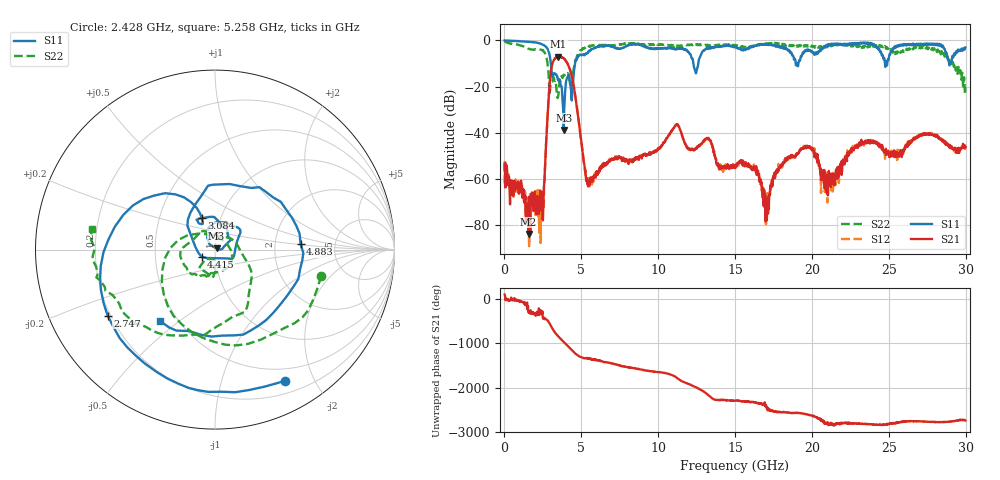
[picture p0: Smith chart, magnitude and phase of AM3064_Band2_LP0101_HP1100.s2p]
# Hz S DB R 50.0
!freq dBS11 angS11 dBS21 angS21 dBS12 angS12 dBS22 angS22
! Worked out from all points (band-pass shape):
!   1600 points, 10 MHz to 29.98 GHz, reference 50 ohm
!   highest |S21| = -7.01 dB at 3.515 GHz (marker M1); lowest = -83.8 dB at 1.566 GHz (marker M2)
!   |S21| within 3 dB of the highest: 3.122 GHz to 4.094 GHz (972 MHz wide, 26.9 % of centre)
!   lowest |S11| = -38.7 dB at 3.852 GHz (marker M3), VSWR 1.02, Z = 50.9 + j0.73 ohm
!   |S11| at or under -10 dB: 3.019 GHz to 4.593 GHz (1.574 GHz wide, 41.4 % of centre); 12.29 GHz to 12.61 GHz (322.1 MHz wide, 2.59 % of centre); 18.95 GHz to 19.12 GHz (176.6 MHz wide, 0.928 % of centre)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
!   |S22| runs from -25.0 to -0.3 dB; largest |S21 - S12| = 0.011
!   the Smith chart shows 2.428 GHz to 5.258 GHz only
!   S11 on the Smith chart (normalised r, x): 2.428 GHz: 0.35, -1.62; 2.747 GHz: 0.19, -0.27; 3.084 GHz: 0.82, +0.30; 4.415 GHz: 0.86, -0.07; 4.883 GHz: 2.81, +0.23; 5.258 GHz: 0.40, -0.43
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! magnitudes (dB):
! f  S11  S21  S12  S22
! 10 MHz  0.0  -53.7  -52.4  -0.3
! 1.566 GHz  -0.6  -83.8  -77.2  -3.6
! 2.428 GHz  -1.6  -65.5  -71.9  -4.3
! 2.747 GHz  -3.1  -40.0  -39.9  -7.7
! 3.084 GHz  -14.5  -10.8  -10.8  -18.0
! 3.515 GHz  -17.3  -7.0  -7.1  -23.1
! 3.852 GHz  -38.7  -7.7  -7.7  -14.9
! 4.415 GHz  -21.4  -16.6  -16.5  -17.9
! 4.883 GHz  -6.4  -38.1  -37.9  -4.9
! 5.015 GHz  -6.5  -44.8  -44.8  -4.3
! 5.258 GHz  -6.0  -56.2  -56.5  -3.2
! 10 GHz  -3.5  -47.2  -46.9  -1.9
! 11.24 GHz  -3.8  -36.5  -36.5  -2.6
! 15 GHz  -2.7  -55.3  -54.7  -2.0
! 16.35 GHz  -2.3  -57.0  -55.5  -2.4
! 17.07 GHz  -2.0  -77.9  -73.3  -1.6
! 17.93 GHz  -2.6  -54.9  -55.3  -1.9
! 19.99 GHz  -4.7  -46.8  -46.6  -2.3
! 21.25 GHz  -1.5  -57.7  -64.8  -2.6
! 23.1 GHz  -1.4  -44.8  -44.3  -2.5
! 25 GHz  -8.1  -49.6  -49.2  -3.2
! 29.98 GHz  -3.1  -46.2  -45.5  -20.2
